TYPE "EN_ServiceID"
VERSION : 0.1


  STRUCT
   UNKNOWN : BYTE ;	//Unknown
   ACYCLIC_READ : BYTE  := B#16#10;	//Acyclic read request
   ACYCLIC_WRITE : BYTE  := B#16#11;	//Acyclic write request
   CYCLIC : BYTE  := B#16#12;	//Cyclic request
  END_STRUCT ;
END_TYPE

